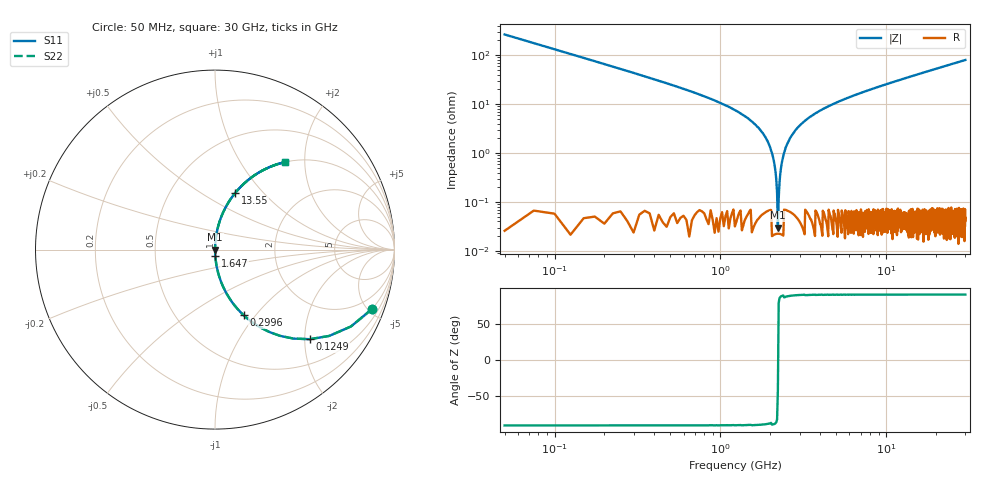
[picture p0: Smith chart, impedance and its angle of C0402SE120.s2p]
!	AVX Thin Film Operation 	Date: April 2014
!	Description: Accu-P® Series, Thin Film  SMD RF Capacitor
!	Part Number: 04023K120FBSTR
# MHZ S MA R 50
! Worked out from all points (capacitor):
!   1201 points, 50 MHz to 30 GHz, reference 50 ohm
!   read as one part in series: C = 12 pF near 199.8 MHz
!   lowest |Z| = 29.8 mohm at 2.221 GHz (marker M1)
!   series resonance near 2.225 GHz, so ESL is about 430 pH
!   S11 on the Smith chart (normalised r, x): 50 MHz: 0.99, -5.30; 124.9 MHz: 1.00, -2.12; 299.6 MHz: 1.00, -0.87; 1.647 GHz: 1.00, -0.07; 13.55 GHz: 1.00, +0.71; 30 GHz: 1.00, +1.60
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50  0.936 -20.7  0.353 69.3  0.353 69.3  0.936 -20.7
124.875  0.727 -43.4  0.687 46.6  0.687 46.6  0.727 -43.4
299.583  0.399 -66.5  0.917 23.5  0.917 23.5  0.399 -66.5
624.042  0.192 -78.8  0.981 11.1  0.981 11.1  0.192 -78.8
1647.333  0.036 -87.2  0.999 2.1  0.999 2.1  0.036 -87.2
1921.875  0.018 -87.5  0.999 1.0  0.999 1.0  0.018 -87.5
2021.708  0.011 -87.1  0.999 0.7  0.999 0.7  0.011 -87.1
2121.542  0.005699 -85.1  1 0.3  1 0.3  0.005699 -85.1
2221.375  0.0004924 -24.0  1 0.0  1 0.0  0.0004924 -24.0
2321.208  0.00506 84.6  1 -0.3  1 -0.3  0.00506 84.6
2446  0.011 87.1  0.999 -0.6  0.999 -0.6  0.011 87.1
2545.833  0.016 87.5  0.999 -0.9  0.999 -0.9  0.016 87.5
2970.125  0.035 87.3  0.999 -2.0  0.999 -2.0  0.035 87.3
3818.708  0.067 85.8  0.997 -3.9  0.997 -3.9  0.067 85.8
5041.667  0.108 83.6  0.994 -6.2  0.994 -6.2  0.108 83.6
7113.208  0.169 80.1  0.985 -9.8  0.985 -9.8  0.169 80.1
10058.29  0.248 75.5  0.968 -14.4  0.968 -14.4  0.248 75.5
13552.46  0.333 70.5  0.943 -19.4  0.943 -19.4  0.333 70.5
15025  0.366 68.5  0.93 -21.5  0.93 -21.5  0.366 68.5
20016.67  0.468 62.1  0.883 -27.9  0.883 -27.9  0.468 62.1
25033.29  0.554 56.3  0.832 -33.6  0.832 -33.6  0.554 56.3
30000  0.624 51.3  0.781 -38.6  0.781 -38.6  0.624 51.3
